(* Logix 5000 Rung export; software revision 16.04 *)

MODULES
   MVI69DFNT : vendor None type None code None
   Local : vendor None type None code None
END_MODULES

TYPE DFNTConnectionInput :   // Connection pin for the Add-On instruction.
STRUCT
   Data : INT[62];   // Add-On data array for connection input pin.
END_STRUCT
END_TYPE

TYPE DFNTSTATUS :   // This status data is returned on each read block and can be used to detect proper module operation.
STRUCT
   PassCnt : INT;   // Program cycle counter
   Product : INT[2];   // Product number
   Rev : INT[2];   // Firmware Revision
   OP : INT[2];   // Operating System revision
   Run : INT[2];   // Run number
   Block : DFNTBlock;   // Block transfer statistics
   Port80Stats : DFNTPort80Status;   // Status of port 80
   ClientStatus : DFNT_ClientStatus;   // Client status data
   DFNTServer : DFNTServerStatus[20];   // MNet server status data
   CommandStatus : DFNTCommandsStatus;   // DFNT Command Status
END_STRUCT
END_TYPE

TYPE DFNTServerStatusBits :   // Control Bits to poll Server status information
STRUCT
   GetServersStat_0_4 : BOOL;   // Server Status Data of Slaves 0 to 4
   GetServersStat_5_9 : BOOL;   // Server Status Data of Slaves 5 to 9
   GetServersStat_10_14 : BOOL;   // Server Status Data of Slaves 10 to 14
   GetServersStat_15_19 : BOOL;   // Server Status Data of Slaves 15 to 19
END_STRUCT
END_TYPE

TYPE DFNT_ClientStatus :   // This object is used to store Client Status.
STRUCT
   CmdReq : INT;   // Total number of command list requests sent
   CmdResp : INT;   // Total number of command list responses received
   CmdErr : INT;   // Total number of command list errors
   Requests : INT;   // Total number of requests for port
   Responses : INT;   // Total number of responses for port
   ErrSent : INT;   // Total number of errors sent
   ErrRec : INT;   // Total number of errors received
   CfgErrWord : INT;   // Configuration Error Word
   CurErr : INT;   // Current Error code
   LastErr : INT;   // Last recorded error code
END_STRUCT
END_TYPE

TYPE DFNTBlock :   // This object is used to store the block transfer statistics for the MVI69-DFNT module.
STRUCT
   Read : INT;   // Total number of read block transfers
   Write : INT;   // Total number of write block transfers
   Parse : INT;   // Total number of blocks parsed
   Event : INT;   // Total number of event blocks received
   Cmd : INT;   // Total number of command blocks received
   Err : INT;   // Total number of block transfer errors
END_STRUCT
END_TYPE

TYPE DFNTDATA :
STRUCT
   ReadData : INT[600];   // Data read from the module to the processor
   WriteData : INT[600];   // Data written from the processor to the module
END_STRUCT
END_TYPE

TYPE DFNTCommandsStatus :   // DFNT CommandsStatus
STRUCT
   CommandStartIndex : INT;   // Index of first command
   CommandCount : INT;   // Number of commands (1 to 50)
   CMDErrorStat : INT[50];   // Array of command error codes
END_STRUCT
END_TYPE

TYPE DFNTCONTROL :   // MVI69-DFNT module control
STRUCT
   BootTimer : TIMER;   // Timer to reset reboot request
   WarmBoot : BOOL;   // Warm Boot
   ColdBoot : BOOL;   // Cold Boot
   ControlBits : DFNTControlBits;   // ControlBits for special command requests
END_STRUCT
END_TYPE

TYPE DFNTServerStatus :   // DFNT Server Status
STRUCT
   SocketState : INT;   // DFNT Server Status
   ConnectionState : INT;   // Connection state
   OpenCount : INT;   // Total number of times the server has performed an open operation.
   EstablishCount : INT;   // Total number of times a connection has been established on the server.
   CloseCount : INT;   // Total number of times the server has performed a close operation.
   ReadCount : INT;   // Total number of packets received by the server.
   MessageCount : INT;   // Total number of message receive by the server.
   WriteCount : INT;   // Total number of packets sent from the server to the client.
   Timeout : INT;   // Total number of times the server as reached a connection timeout condition.
   HostPort : INT;   // Service port on client connected to the server.
   HostIPAddr : INT[2];   // IP address of the client connected to the server.
END_STRUCT
END_TYPE

TYPE DFNTControlBits :   // DFNT ControlBits
STRUCT
   EnableCommands : BOOL;   // Dynamically enables configured commands (enable code = 1)
   DisableCommands : BOOL;   // Dynamically disables configured commands (enable code = 0)
   ConditionalCommands : BOOL;   // Dynamically sets configured commands as conditional (enable code = 2)
   GetServersStat : DFNTServerStatusBits;   // Retrieves server status
   GetModuleStat : BOOL;   // Retrieves module status
   StatusCommandErr : BOOL;   // Retrieves command errors
END_STRUCT
END_TYPE

TYPE DFNTUTIL :   // Internal ladder usage - should not be accessed by user application
STRUCT
   ReadDataSizeGet : INT;   // Gets ReadData Array Length.
   WriteDataSizeGet : INT;   // Gets WriteData Array Length.
   ReadDataBlkCount : INT;   // holds the value of the Block Counts of the Read Data Array.
   WriteDataBlkCount : INT;   // holds the value of the Block Counts of the Write Data Array.
   RBTSremainder : INT;   // The remainder of the 60, 120 or 240 block to transfer.
   WBTSremainder : INT;   // The remainder of the 60, 120 or 240 block to transfer.
   LastRead : INT;   // Backplane last read
   LastWrite : INT;   // Backplane last write
   BlockIndex : INT;   // Block index
END_STRUCT
END_TYPE

TYPE DFNTCONFIG :   // MVI69-MCM block transfer size configuration.
STRUCT
   BlockTransferSize : INT;   // This value should be 60, 120 or 240 words. Needs to match Module's backplane Connection Parameters.
END_STRUCT
END_TYPE

TYPE DFNTModuleDef :   // DFNT ModuleDef
STRUCT
   CONFIG : DFNTCONFIG;   // Configuration information
   DATA : DFNTDATA;   // DFNT data transferred between module and processor
   STATUS : DFNTSTATUS;   // Status information in each read block
   CONTROL : DFNTCONTROL;   // Optional requests from the processor to the module
   UTIL : DFNTUTIL;   // Used only internally for ladder processing
END_STRUCT
END_TYPE

TYPE DFNTPort80Status :   // DFNT Port 80 Status
STRUCT
   No_of_Requests : INT;   // Total Number of HTTP requests for the module
   No_of_Responses : INT;   // Total Number of HTTP response Messages generated
END_STRUCT
END_TYPE

TYPE DFNTConnectionOutput :   // Connection pin for the Add-On instruction.
STRUCT
   Data : INT[61];   // Add-On data array for connection output pin.
END_STRUCT
END_TYPE

ADD_ON_INSTRUCTION AOI69DFNT   (* revision 1.4, vendor Prosoft Technology Inc. *)
// Add-On for the MVI69-DFNT module.
// Revision note:
// v1.2 - re-exported AOI rung
// v1.3 - Fix to ServerStatus Functionality
// v1.4 - Fixed Boot Loop issue found when rebooting
VAR_IN_OUT
   Connection_Input : DFNTConnectionInput; {required}
   Connection_Output : DFNTConnectionOutput; {required}
   DFNT : DFNTModuleDef; {required}
END_VAR

ROUTINE Logic   (* ladder *)
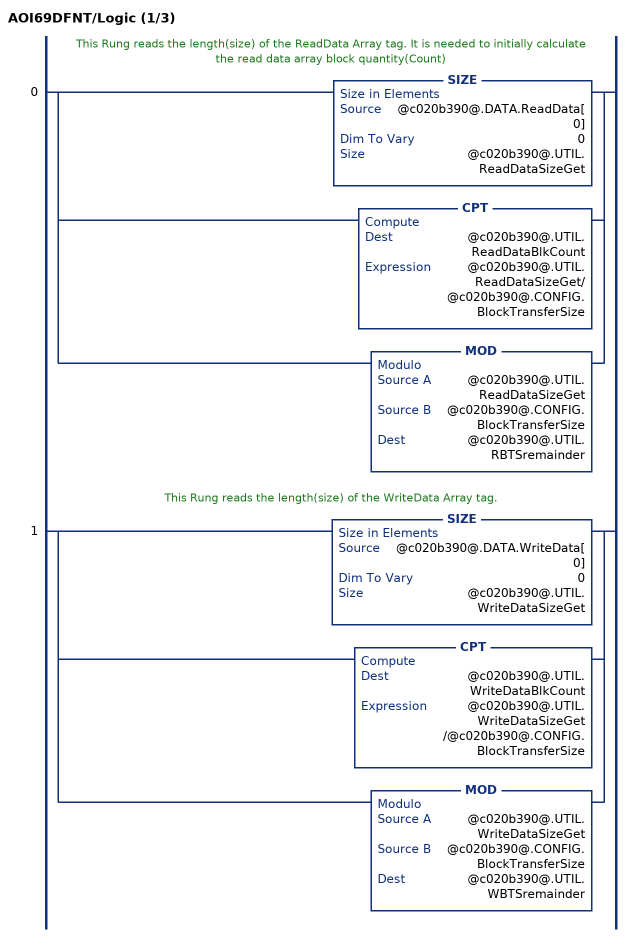
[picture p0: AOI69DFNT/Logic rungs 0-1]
   // This Rung reads the length(size) of the ReadData Array tag. It is needed to initially calculate the read data array block quantity(Count)
   0: [SIZE(@c020b390@.DATA.ReadData[0],0,@c020b390@.UTIL.ReadDataSizeGet) ,CPT(@c020b390@.UTIL.ReadDataBlkCount,@c020b390@.UTIL.ReadDataSizeGet/@c020b390@.CONFIG.BlockTransferSize) ,MOD(@c020b390@.UTIL.ReadDataSizeGet,@c020b390@.CONFIG.BlockTransferSize,@c020b390@.UTIL.RBTSremainder) ];
   // This Rung reads the length(size) of the WriteData Array tag.
   1: [SIZE(@c020b390@.DATA.WriteData[0],0,@c020b390@.UTIL.WriteDataSizeGet) ,CPT(@c020b390@.UTIL.WriteDataBlkCount,@c020b390@.UTIL.WriteDataSizeGet /@c020b390@.CONFIG.BlockTransferSize) ,MOD(@c020b390@.UTIL.WriteDataSizeGet,@c020b390@.CONFIG.BlockTransferSize,@c020b390@.UTIL.WBTSremainder) ];
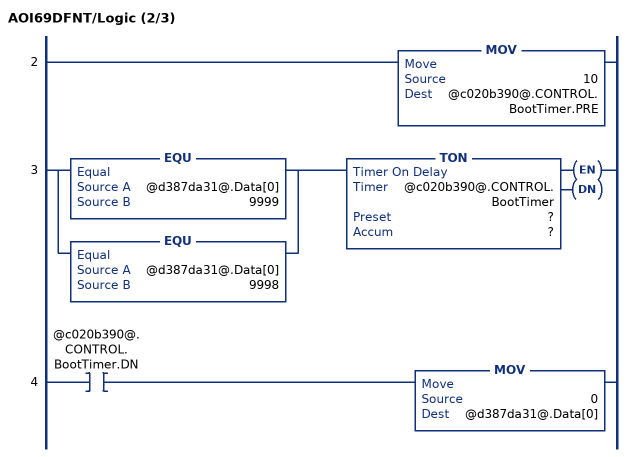
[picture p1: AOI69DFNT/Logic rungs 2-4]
   2: MOV(10,@c020b390@.CONTROL.BootTimer.PRE);
   3: [EQU(@d387da31@.Data[0],9999) ,EQU(@d387da31@.Data[0],9998) ]TON(@c020b390@.CONTROL.BootTimer,?,?);
   4: XIC(@c020b390@.CONTROL.BootTimer.DN)MOV(0,@d387da31@.Data[0]);
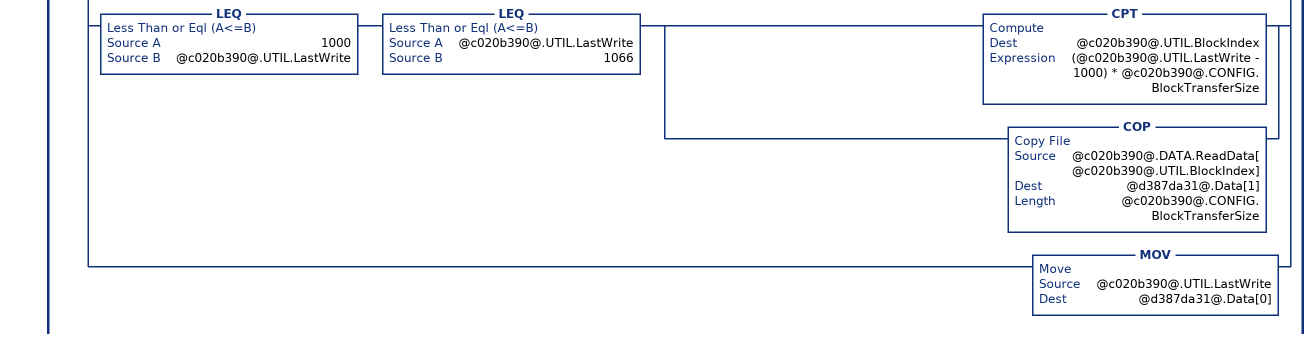
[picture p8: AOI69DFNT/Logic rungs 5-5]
   // The routines will only be scanned once the processor receives a new read block ID from the module
   5: NEQ(@c020b390@.UTIL.LastRead,@46f1db06@.Data[0])[MOV(@46f1db06@.Data[0],@c020b390@.UTIL.LastRead) ,GEQ(@c020b390@.UTIL.LastRead,1) [LEQ(@c020b390@.UTIL.LastRead,@c020b390@.UTIL.ReadDataBlkCount) [CPT(@c020b390@.UTIL.BlockIndex,(@c020b390@.UTIL.LastRead - 1) * @c020b390@.CONFIG.BlockTransferSize) ,COP(@46f1db06@.Data[2],@c020b390@.DATA.ReadData[@c020b390@.UTIL.BlockIndex],@c020b390@.CONFIG.BlockTransferSize) ] ,CMP(@c020b390@.UTIL.LastRead - @c020b390@.UTIL.ReadDataBlkCount = 1) GRT(@c020b390@.UTIL.RBTSremainder,0) [CPT(@c020b390@.UTIL.BlockIndex,(@c020b390@.UTIL.LastRead - 1) * @c020b390@.CONFIG.BlockTransferSize) ,COP(@46f1db06@.Data[2],@c020b390@.DATA.ReadData[@c020b390@.UTIL.BlockIndex],@c020b390@.UTIL.RBTSremainder) ] ] ,[EQU(@c020b390@.UTIL.LastRead,-1) ,EQU(@c020b390@.UTIL.LastRead,0) ,EQU(@c020b390@.UTIL.LastRead,250) ] [COP(@46f1db06@.Data[2],@c020b390@.STATUS.PassCnt,1) ,COP(@46f1db06@.Data[3],@c020b390@.STATUS.Product[0],2) ,COP(@46f1db06@.Data[5],@c020b390@.STATUS.Rev[0],2) ,COP(@46f1db06@.Data[7],@c020b390@.STATUS.OP[0],2) ,COP(@46f1db06@.Data[9],@c020b390@.STATUS.Run[0],2) ,COP(@46f1db06@.Data[31],@c020b390@.STATUS.Block.Read,6) ,COP(@46f1db06@.Data[14],@c020b390@.STATUS.Port80Stats.No_of_Requests,2) ,COP(@46f1db06@.Data[21],@c020b390@.STATUS.ClientStatus.CmdReq,10) ] ,EQU(@c020b390@.UTIL.LastRead,2000) [COP(@46f1db06@.Data[2],@c020b390@.STATUS.CommandStatus.CMDErrorStat[0],50) ,OTU(@c020b390@.CONTROL.ControlBits.StatusCommandErr) ] ,EQU(@c020b390@.UTIL.LastRead,251) [COP(@46f1db06@.Data[2],@c020b390@.STATUS.DFNTServer[0].SocketState,60) ,OTU(@c020b390@.CONTROL.ControlBits.GetServersStat.GetServersStat_0_4) ] ,EQU(@c020b390@.UTIL.LastRead,252) [COP(@46f1db06@.Data[2],@c020b390@.STATUS.DFNTServer[5].SocketState,60) ,OTU(@c020b390@.CONTROL.ControlBits.GetServersStat.GetServersStat_5_9) ] ,EQU(@c020b390@.UTIL.LastRead,253) [COP(@46f1db06@.Data[2],@c020b390@.STATUS.DFNTServer[10].SocketState,60) ,OTU(@c020b390@.CONTROL.ControlBits.GetServersStat.GetServersStat_10_14) ] ,EQU(@c020b390@.UTIL.LastRead,254) [COP(@46f1db06@.Data[2],@c020b390@.STATUS.DFNTServer[15].SocketState,60) ,OTU(@c020b390@.CONTROL.ControlBits.GetServersStat.GetServersStat_15_19) ] ,MOV(@46f1db06@.Data[1],@c020b390@.UTIL.LastWrite) ,XIC(@c020b390@.CONTROL.ColdBoot) NEQ(@c020b390@.UTIL.LastRead,0) [MOV(9999,@c020b390@.UTIL.LastWrite) ,OTU(@c020b390@.CONTROL.ColdBoot) ] ,XIC(@c020b390@.CONTROL.WarmBoot) NEQ(@c020b390@.UTIL.LastRead,0) [MOV(9998,@c020b390@.UTIL.LastWrite) ,OTU(@c020b390@.CONTROL.WarmBoot) ] ,GEQ(@c020b390@.UTIL.LastWrite,1) [LEQ(@c020b390@.UTIL.LastWrite,@c020b390@.UTIL.WriteDataBlkCount) [CPT(@c020b390@.UTIL.BlockIndex,(@c020b390@.UTIL.LastWrite - 1) * @c020b390@.CONFIG.BlockTransferSize) ,COP(@c020b390@.DATA.WriteData[@c020b390@.UTIL.BlockIndex],@d387da31@.Data[1],@c020b390@.CONFIG.BlockTransferSize) ] ,CMP(@c020b390@.UTIL.LastWrite - @c020b390@.UTIL.WriteDataBlkCount = 1) GRT(@c020b390@.UTIL.WBTSremainder,0) [CPT(@c020b390@.UTIL.BlockIndex,(@c020b390@.UTIL.LastWrite - 1) * @c020b390@.CONFIG.BlockTransferSize) ,COP(@c020b390@.DATA.WriteData[@c020b390@.UTIL.BlockIndex],@d387da31@.Data[1],@c020b390@.UTIL.WBTSremainder) ] ] ,XIC(@c020b390@.CONTROL.ControlBits.StatusCommandErr) [MOV(2000,@c020b390@.UTIL.LastWrite) ,MOV(@c020b390@.STATUS.CommandStatus.CommandStartIndex,@d387da31@.Data[1]) ,MOV(@c020b390@.STATUS.CommandStatus.CommandCount,@d387da31@.Data[2]) ,OTL(@c020b390@.CONTROL.ControlBits.StatusCommandErr) ] ,XIC(@c020b390@.CONTROL.ControlBits.DisableCommands) [MOV(@c020b390@.STATUS.CommandStatus.CommandCount,@d387da31@.Data[1]) ,MOV(@c020b390@.STATUS.CommandStatus.CommandStartIndex,@d387da31@.Data[2]) ,MOV(3000,@c020b390@.UTIL.LastWrite) ,OTU(@c020b390@.CONTROL.ControlBits.DisableCommands) ] ,XIC(@c020b390@.CONTROL.ControlBits.EnableCommands) [MOV(@c020b390@.STATUS.CommandStatus.CommandCount,@d387da31@.Data[1]) ,MOV(@c020b390@.STATUS.CommandStatus.CommandStartIndex,@d387da31@.Data[2]) ,MOV(3001,@c020b390@.UTIL.LastWrite) ,OTU(@c020b390@.CONTROL.ControlBits.EnableCommands) ] ,XIC(@c020b390@.CONTROL.ControlBits.ConditionalCommands) [MOV(@c020b390@.STATUS.CommandStatus.CommandCount,@d387da31@.Data[1]) ,MOV(@c020b390@.STATUS.CommandStatus.CommandStartIndex,@d387da31@.Data[2]) ,MOV(3002,@c020b390@.UTIL.LastWrite) ,OTU(@c020b390@.CONTROL.ControlBits.ConditionalCommands) ] ,XIC(@c020b390@.CONTROL.ControlBits.GetModuleStat) [MOV(250,@c020b390@.UTIL.LastWrite) ,OTU(@c020b390@.CONTROL.ControlBits.GetModuleStat) ] ,XIC(@c020b390@.CONTROL.ControlBits.GetServersStat.GetServersStat_0_4) [MOV(251,@c020b390@.UTIL.LastWrite) ,OTL(@c020b390@.CONTROL.ControlBits.GetServersStat.GetServersStat_0_4) ] ,XIC(@c020b390@.CONTROL.ControlBits.GetServersStat.GetServersStat_5_9) [MOV(252,@c020b390@.UTIL.LastWrite) ,OTL(@c020b390@.CONTROL.ControlBits.GetServersStat.GetServersStat_5_9) ] ,XIC(@c020b390@.CONTROL.ControlBits.GetServersStat.GetServersStat_10_14) [MOV(253,@c020b390@.UTIL.LastWrite) ,OTL(@c020b390@.CONTROL.ControlBits.GetServersStat.GetServersStat_10_14) ] ,XIC(@c020b390@.CONTROL.ControlBits.GetServersStat.GetServersStat_15_19) [MOV(254,@c020b390@.UTIL.LastWrite) ,OTL(@c020b390@.CONTROL.ControlBits.GetServersStat.GetServersStat_15_19) ] ,LEQ(1000,@c020b390@.UTIL.LastWrite) LEQ(@c020b390@.UTIL.LastWrite,1066) [CPT(@c020b390@.UTIL.BlockIndex,(@c020b390@.UTIL.LastWrite - 1000) * @c020b390@.CONFIG.BlockTransferSize) ,COP(@c020b390@.DATA.ReadData[@c020b390@.UTIL.BlockIndex],@d387da31@.Data[1],@c020b390@.CONFIG.BlockTransferSize) ] ,MOV(@c020b390@.UTIL.LastWrite,@d387da31@.Data[0]) ];
END_ROUTINE
END_ADD_ON_INSTRUCTION

VAR_GLOBAL   (* controller tags *)
   Local:1:O : AB:1769_MODULE_INT_122Bytes:O:0;
   DFNT : DFNTModuleDef;
   Local:1:I : AB:1769_MODULE_INT_128Bytes:I:0;
   Connection_Input : DFNTConnectionInput;
   AOI69DFNT : AOI69DFNT;
   Connection_Output : DFNTConnectionOutput;
END_VAR

PROGRAM MainProgram

ROUTINE MainRoutine   (* ladder *)
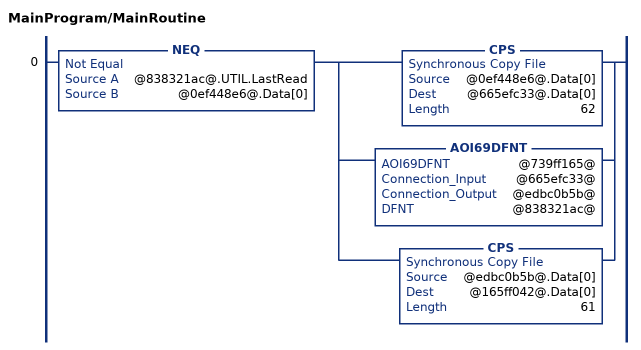
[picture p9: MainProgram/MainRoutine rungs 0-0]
   0: NEQ(@838321ac@.UTIL.LastRead,@0ef448e6@.Data[0])[CPS(@0ef448e6@.Data[0],@665efc33@.Data[0],62) ,AOI69DFNT(@739ff165@,@665efc33@,@edbc0b5b@,@838321ac@) ,CPS(@edbc0b5b@.Data[0],@165ff042@.Data[0],61) ];
END_ROUTINE
END_PROGRAM
